(* Logix 5000 AddOnInstructionDefinition export OM_AZ_WRITE; software revision 30.00 *)

ADD_ON_INSTRUCTION OM_AZ_WRITE   (* revision 1.3, vendor ORIENTALMOTOR CO.,LTD. *)
// Revision note:
// Implicit message based on AZD-AEP,-CEP and -KEP.
// Help:
// This AOI is used to write data from the scanner to the driver via Implicit communication.
VAR_IN_OUT
   ImplicitMSGinput : INT[28]; {required}   // Implicit message Input (driver->scanner)
        [0]   // Remote I/O (R-OUT)
        [0].0   // R-OUT0
        [0].1   // R-OUT1
        [0].2   // R-OUT2
        [0].3   // R-OUT3
        [0].4   // R-OUT4
        [0].5   // R-OUT5
        [0].6   // R-OUT6
        [0].7   // R-OUT7
        [0].8   // R-OUT8
        [0].9   // R-OUT9
        [0].10   // R-OUT10
        [0].11   // R-OUT11
        [0].12   // R-OUT12
        [0].13   // R-OUT13
        [0].14   // R-OUT14
        [0].15   // R-OUT15
        [1]   // Operation data number selection_R
        [1].0   // M0_R
        [1].1   // M1_R
        [1].2   // M2_R
        [1].3   // M3_R
        [1].4   // M4_R
        [1].5   // M5_R
        [1].6   // M6_R
        [1].7   // M7_R
        [1].8   // Reserved
        [1].9   // Reserved
        [1].10   // Reserved
        [1].11   // Reserved
        [1].12   // Reserved
        [1].13   // Reserved
        [1].14   // Reserved
        [1].15   // Reserved
        [2]   // Fixed I/O (OUT)
        [2].0   // SEQ-BSY
        [2].1   // MOVE
        [2].2   // IN-POS
        [2].3   // START_R
        [2].4   // HOME-END
        [2].5   // READY
        [2].6   // DCMD-RDY
        [2].7   // ALM-A
        [2].8   // TRIG_R
        [2].9   // TRIG-MODE_R
        [2].10   // SET-ERR
        [2].11   // EXE-ERR
        [2].12   // DCMD-FULL
        [2].13   // STOP_R
        [2].14   // ETO-MON
        [2].15   // TLC
        [3]   // Present alarm
        [4]   // Feedback position (lower)
        [5]   // Feedback position (upper)
        [6]   // Feedback speed [Hz] (lower)
        [7]   // Feedback speed [Hz] (upper)
        [8]   // Command position (lower)
        [9]   // Command position (upper)
        [10]   // Torque monitor
        [11]   // CST operating current
        [12]   // Information (lower)
        [13]   // Information (upper)
        [14]   // Reserved
        [15]   // Read parameter ID_R
        [16]   // Read/write status
        [16].0   // Reserved
        [16].1   // Reserved
        [16].2   // Reserved
        [16].3   // Reserved
        [16].4   // Reserved
        [16].5   // Reserved
        [16].6   // Reserved
        [16].7   // RD-ERR
        [16].8   // WR-END
        [16].9   // SYS-BSY
        [16].10   // Reserved
        [16].11   // WR-SET-ERR
        [16].12   // WR-IF-ERR
        [16].13   // WR-NV-ERR
        [16].14   // WR-EXE-ERR
        [16].15   // WR-ERR
        [17]   // Write parameter ID_R
        [18]   // Read data (lower)
        [19]   // Read data (upper)
        [20]   // Assignable monitor 0 (lower)
        [21]   // Assignable monitor 0 (upper)
        [22]   // Assignable monitor 1 (lower)
        [23]   // Assignable monitor 1 (upper)
        [24]   // Assignable monitor 2 (lower)
        [25]   // Assignable monitor 2 (upper)
        [26]   // Assignable monitor 3 (lower)
        [27]   // Assignable monitor 3 (upper)
   ImplicitMSGoutput : INT[20]; {required}   // Implicit message Output (scanner->driver)
        [0]   // Remote I/O(R-IN)
        [0].0   // R-IN0
        [0].1   // R-IN1
        [0].2   // R-IN2
        [0].3   // R-IN3
        [0].4   // R-IN4
        [0].5   // R-IN5
        [0].6   // R-IN6
        [0].7   // R-IN7
        [0].8   // R-IN8
        [0].9   // R-IN9
        [0].10   // R-IN10
        [0].11   // R-IN11
        [0].12   // R-IN12
        [0].13   // R-IN13
        [0].14   // R-IN14
        [0].15   // R-IN15
        [1]   // Operation data number selection
        [1].0   // M0
        [1].1   // M1
        [1].2   // M2
        [1].3   // M3
        [1].4   // M4
        [1].5   // M5
        [1].6   // M6
        [1].7   // M7
        [1].8   // Reserved
        [1].9   // Reserved
        [1].10   // Reserved
        [1].11   // Reserved
        [1].12   // Reserved
        [1].13   // Reserved
        [1].14   // Reserved
        [1].15   // Reserved
        [2]   // Fixed I/O(IN)
        [2].0   // FW-JOG
        [2].1   // RV-JOG
        [2].2   // Reserved
        [2].3   // START
        [2].4   // ZHOME
        [2].5   // STOP
        [2].6   // FREE
        [2].7   // ALM-RST
        [2].8   // TRIG
        [2].9   // TRIG-MODE
        [2].10   // ETO-CLR
        [2].11   // Reserved
        [2].12   // FW-JOG-P
        [2].13   // RV-JOG-P
        [2].14   // FW-POS
        [2].15   // RV-POS
        [3]   // Direct data operation operation type
        [4]   // Direct data operation position (lower)
        [5]   // Direct data operation position (upper)
        [6]   // Direct data operation operating speed (lower)
        [7]   // Direct data operation operating speed (upper)
        [8]   // Direct data operation starting/changing rate (lower)
        [9]   // Direct data operation starting/changing rate (upper)
        [10]   // Direct data operation stopping deceleration (lower)
        [11]   // Direct data operation stopping deceleration (upper)
        [12]   // Direct data operation operating current
        [13]   // Direct data operation forwarding destination
        [14]   // Reserved
        [15]   // Read parameter ID
        [16]   // Write request
        [16].0   // WR-REQ
        [16].1   // Reserved
        [16].2   // Reserved
        [16].3   // Reserved
        [16].4   // Reserved
        [16].5   // Reserved
        [16].6   // Reserved
        [16].7   // Reserved
        [16].8   // Reserved
        [16].9   // Reserved
        [16].10   // Reserved
        [16].11   // Reserved
        [16].12   // Reserved
        [16].13   // Reserved
        [16].14   // Reserved
        [16].15   // Reserved
        [17]   // Write parameter ID
        [18]   // Write data (lower)
        [19]   // Write data (upper)
END_VAR
VAR_INPUT
   Set_Exe : BOOL; {visible}   // Execute AOI
   WritePRMID : INT; {visible}   // Write parameter ID
   WriteData : DINT; {visible}   // Write data
END_VAR
VAR_OUTPUT
   Sts_Busy : BOOL; {access None, visible}   // Executing status in AOI
   Sts_Err : BOOL; {access None, visible}   // Error status in AOI
   Sts_Done : BOOL; {access None, visible}   // Complete status in AOI
END_VAR
VAR
   flag_Ini : BOOL; {access None}
   flag_Ready : BOOL; {access None}
   WRITE_REQUEST : INT := 1; {access None}
   Read_WriteStatus : INT; {access None}   // Read/write status
        .0   // Reserved
        .1   // Reserved
        .2   // Reserved
        .3   // Reserved
        .4   // Reserved
        .5   // Reserved
        .6   // Reserved
        .7   // RD-ERR
        .8   // WR-END
        .9   // SYS-BSY
        .10   // Reserved
        .11   // WR-SET-ERR
        .12   // WR-IF-ERR
        .13   // WR-NV-ERR
        .14   // WR-EXE-ERR
        .15   // WR-ERR
   flag_End : BOOL; {access None}
END_VAR

ROUTINE Logic   (* ladder *)
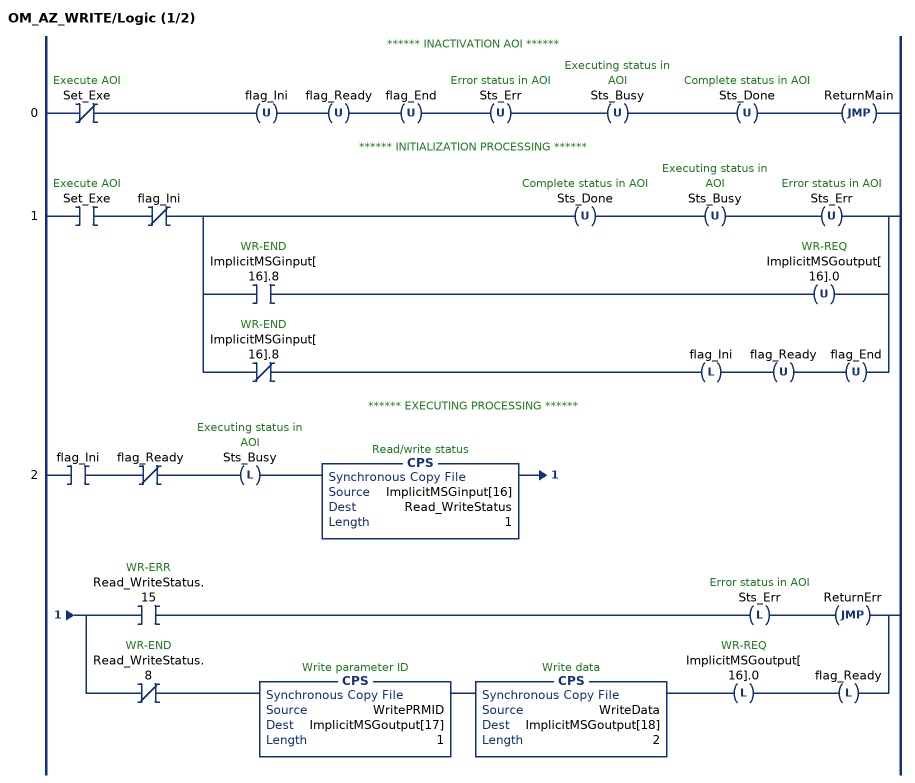
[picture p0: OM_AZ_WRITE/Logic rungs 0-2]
   // ****** INACTIVATION AOI ******
   0: XIO(Set_Exe)OTU(flag_Ini)OTU(flag_Ready)OTU(flag_End)OTU(Sts_Err)OTU(Sts_Busy)OTU(Sts_Done)JMP(ReturnMain);
   // ****** INITIALIZATION PROCESSING ******
   1: XIC(Set_Exe)XIO(flag_Ini)[OTU(Sts_Done) OTU(Sts_Busy) OTU(Sts_Err) ,[XIC(ImplicitMSGinput[16].8) OTU(ImplicitMSGoutput[16].0) ,XIO(ImplicitMSGinput[16].8) OTL(flag_Ini) OTU(flag_Ready) OTU(flag_End) ] ];
   // ****** EXECUTING PROCESSING ******
   2: XIC(flag_Ini)XIO(flag_Ready)OTL(Sts_Busy)CPS(ImplicitMSGinput[16],Read_WriteStatus,1)[XIC(Read_WriteStatus.15) OTL(Sts_Err) JMP(ReturnErr) ,XIO(Read_WriteStatus.8) CPS(WritePRMID,ImplicitMSGoutput[17],1) CPS(WriteData,ImplicitMSGoutput[18],2) OTL(ImplicitMSGoutput[16].0) OTL(flag_Ready) ];
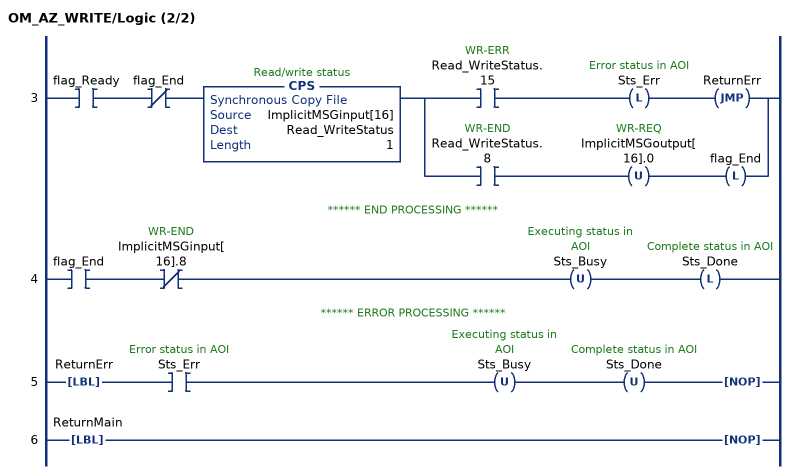
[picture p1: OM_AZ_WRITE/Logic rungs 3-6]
   3: XIC(flag_Ready)XIO(flag_End)CPS(ImplicitMSGinput[16],Read_WriteStatus,1)[XIC(Read_WriteStatus.15) OTL(Sts_Err) JMP(ReturnErr) ,XIC(Read_WriteStatus.8) OTU(ImplicitMSGoutput[16].0) OTL(flag_End) ];
   // ****** END PROCESSING ******
   4: XIC(flag_End)XIO(ImplicitMSGinput[16].8)OTU(Sts_Busy)OTL(Sts_Done);
   // ****** ERROR PROCESSING ******
   5: LBL(ReturnErr)XIC(Sts_Err)OTU(Sts_Busy)OTU(Sts_Done)NOP();
   6: LBL(ReturnMain)NOP();
END_ROUTINE
END_ADD_ON_INSTRUCTION
